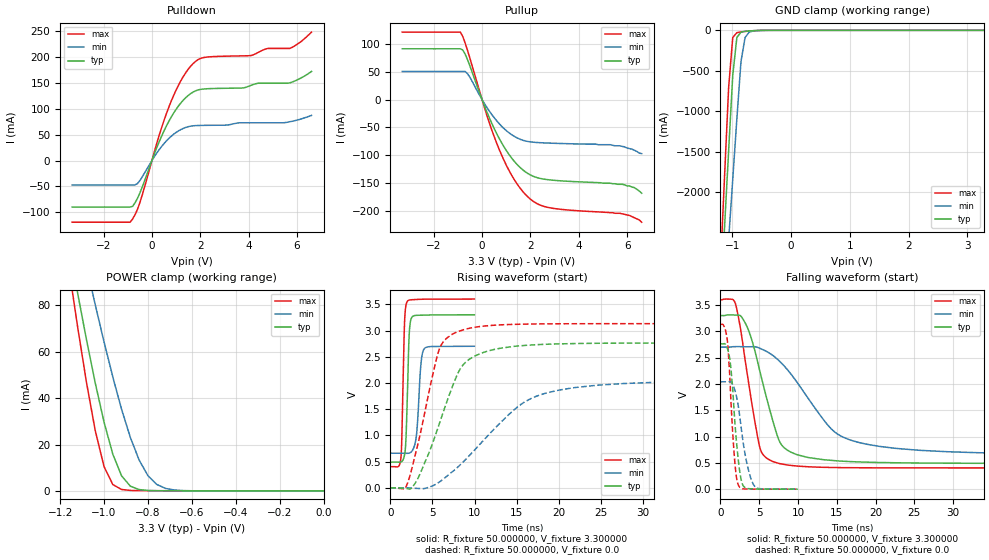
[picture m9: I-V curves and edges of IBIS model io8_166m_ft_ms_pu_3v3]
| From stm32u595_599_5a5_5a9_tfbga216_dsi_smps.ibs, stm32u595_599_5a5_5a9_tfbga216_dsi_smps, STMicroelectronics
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|   Model io8_166m_ft_ms_pu_3v3
[Model]  io8_166m_ft_ms_pu_3v3
Model_type I/O
Polarity   Non-Inverting
Enable   Active-Low
Vinl =   0.990000V
Vinh =   2.310000V
Vmeas =  1.650000V
Cref =   50.000000pF
Rref =   100.000000M
Vref =   0.0V
C_comp   3.517200pF   3.489400pF   3.557800pF
[Temperature Range]   25.000000   0.140000k   -40.000000
[Pullup Reference]   3.300000V   2.700000V   3.600000V
[Pulldown Reference]   0.0V   0.0V   0.0V
[POWER Clamp Reference]   3.300000V   2.700000V   3.600000V
[GND Clamp Reference]   0.0V   0.0V   0.0V
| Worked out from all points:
|   slope of the pulldown table from 0 to 0.495 V, typ, clamps not added: 8.73 ohm
|   slope of the pullup table from 0 to 0.495 V, typ, clamps not added: 9.64 ohm
|   GND clamp passes 1 mA (typ) near -0.50 V on its own axis
|   POWER clamp passes 1 mA (typ) near -0.85 V on its own axis
|   rising waveform, R_fixture 50.000000, V_fixture 3.300000: 20-80 % time 305ps typ, 453ps min, 270ps max; typ from 0.49 V to 3.3 V
|   rising waveform, R_fixture 50.000000, V_fixture 0.0: 20-80 % time 3.81ns typ, 7.79ns min, 2.6ns max; typ from 0.001 V to 2.76 V
|   falling waveform, R_fixture 50.000000, V_fixture 3.300000: 20-80 % time 3.02ns typ, 6.39ns min, 2.05ns max; typ from 3.3 V to 0.49 V
|   falling waveform, R_fixture 50.000000, V_fixture 0.0: 20-80 % time 902ps typ, 1.3ns min, 737ps max; typ from 2.76 V to 0.001 V
[Pulldown]
|Voltage   I(typ)   I(min)   I(max)
-3.3V     -89.71mA   -47.06mA   -119mA
-900mV    -89.71mA   -47.06mA   -119mA
-500mV    -62.92mA   -38.72mA   -81.44mA
300mV     36.2mA     21.01mA    48.7mA
800mV     84.07mA    46.96mA    114.8mA
1.3V      116.7mA    62.09mA    162.4mA
1.8V      134.4mA    67.39mA    191.2mA
2.3V      138.6mA    67.98mA    199.8mA
4.1V      145.2mA    72.76mA    202.7mA
4.8V      149.3mA    72.76mA    216.4mA
5.7V      149.8mA    74.9mA     216.4mA
6.6V      172mA      87.1mA     247.9mA
[Pullup]
|Voltage   I(typ)   I(min)   I(max)
-3.3V     91.1mA     50.4mA     121mA
-900mV    91.1mA     50.4mA     121mA
-800mV    88.97mA    50.4mA     113.5mA
-600mV    71.53mA    46.27mA    88.1mA
200mV     -22.26mA   -14.13mA   -28.38mA
700mV     -69mA      -42.82mA   -88.5mA
1.3V      -109.1mA   -65.19mA   -141.4mA
2V        -135.3mA   -75.91mA   -178.7mA
2.9V      -144.6mA   -78.33mA   -194.9mA
5.8V      -152mA     -84mA      -205mA
6.3V      -158mA     -91mA      -212mA
6.6V      -168mA     -97mA      -220mA
[GND_clamp]
|Voltage   I(typ)   I(min)   I(max)
-3.3V     -9.098A    -9.372A    -9.671A
-1.2V     -3.386A    -4.091A    -2.933A
-1.13V    -2.437A    -3.34A     -1.815A
-1.06V    -1.49A     -2.588A    -705.6mA
-990mV    -555.7mA   -1.839A    -89.03mA
-920mV    -88.12mA   -1.093A    -28.78mA
-850mV    -22.35mA   -387.4mA   -19.84mA
-780mV    -12.12mA   -88.01mA   -13.88mA
-710mV    -7.71mA    -22.52mA   -8.846mA
-640mV    -4.545mA   -7.864mA   -4.87mA
-360mV    -31.12uA   -173.5uA   -8.497uA
3.28V     0A         14.15nA    -7.901nA
[POWER_clamp]
|Voltage   I(typ)   I(min)   I(max)
-3.28V    1.355A     1.167A     1.665A
-1.16V    105.8mA    131.6mA    95.87mA
-1.12V    85.08mA    114mA      70.45mA
-1.08V    65.17mA    96.88mA    46.74mA
-1.04V    46.48mA    80.2mA     25.96mA
-1V       29.63mA    64.18mA    10.49mA
-960mV    15.81mA    49.06mA    2.743mA
-920mV    6.481mA    35.16mA    612.1uA
-840mV    577.5uA    13.29mA    137.6uA
-760mV    93.73uA    2.807mA    97.77uA
-640mV    40.05uA    158.9uA    59.33uA
0V        0A         19.33nA    0A
[Ramp]
| variable   typ   min   max
dV/dt_r  1.65687/3.80732n   1.22412/7.78033n   1.87825/2.59543n
dV/dt_f  1.68570/3.01118n   1.22217/6.37676n   1.91753/2.04585n
R_load = 50.000000
[Rising Waveform]
R_fixture= 50.000000
V_fixture= 3.300000
V_fixture_min= 2.700000
V_fixture_max= 3.600000
|time   V(typ)   V(min)   V(max)
0s        490.5mV    660.4mV    404.1mV
1.261ns   491.5mV    660.4mV    573.4mV
1.682ns   623.2mV    660.2mV    3.106V
1.982ns   1.518V     659mV      3.546V
2.242ns   2.92V      662.6mV    3.581V
2.583ns   3.258V     703.1mV    3.587V
3.103ns   3.29V      1.001V     3.592V
3.604ns   3.292V     2.3V       3.596V
3.964ns   3.293V     2.638V     3.597V
9.97ns    3.3V       2.7V       3.6V
[Rising Waveform]
R_fixture= 50.000000
V_fixture= 0.0
V_fixture_min= 0.0
V_fixture_max= 0.0
|time   V(typ)   V(min)   V(max)
0s        562.9uV    600.6uV    581.8uV
1.802ns   -12.48mV   778.8uV    -1.597mV
3.003ns   101.2mV    -9.126mV   658.4mV
5.886ns   1.256V     118.8mV    2.672V
7.928ns   2.153V     383.4mV    2.974V
8.769ns   2.368V     514.6mV    3.019V
11.05ns   2.583V     905.2mV    3.084V
15.26ns   2.706V     1.564V     3.12V
20.06ns   2.745V     1.866V     3.129V
59.82ns   2.762V     2.041V     3.131V
[Falling Waveform]
R_fixture= 50.000000
V_fixture= 3.300000
V_fixture_min= 2.700000
V_fixture_max= 3.600000
|time   V(typ)   V(min)   V(max)
0s        3.3V       2.7V       3.6V
1.922ns   3.309V     2.709V     3.533V
3.483ns   3.072V     2.707V     2.169V
5.045ns   2.267V     2.68V      814.3mV
6.727ns   1.316V     2.546V     527.7mV
7.688ns   889.5mV    2.424V     485.1mV
9.129ns   700.6mV    2.182V     451.6mV
14.29ns   548.1mV    1.146V     412.9mV
18.14ns   516.7mV    877.8mV    407.3mV
59.82ns   490.5mV    660.4mV    404.1mV
[Falling Waveform]
R_fixture= 50.000000
V_fixture= 0.0
V_fixture_min= 0.0
V_fixture_max= 0.0
|time   V(typ)   V(min)   V(max)
0s        2.762V     2.041V     3.131V
800.8ps   2.714V     2.041V     2.924V
1.201ns   2.483V     2.046V     2.167V
1.542ns   1.992V     2V         1.18V
1.822ns   1.367V     1.9V       579.5mV
2.342ns   509.8mV    1.546V     69.45mV
2.943ns   65.6mV     880.7mV    7.558mV
3.584ns   11.72mV    384.6mV    3.156mV
4.364ns   4.498mV    65.78mV    1.894mV
9.97ns    562.9uV    600.6uV    581.8uV
